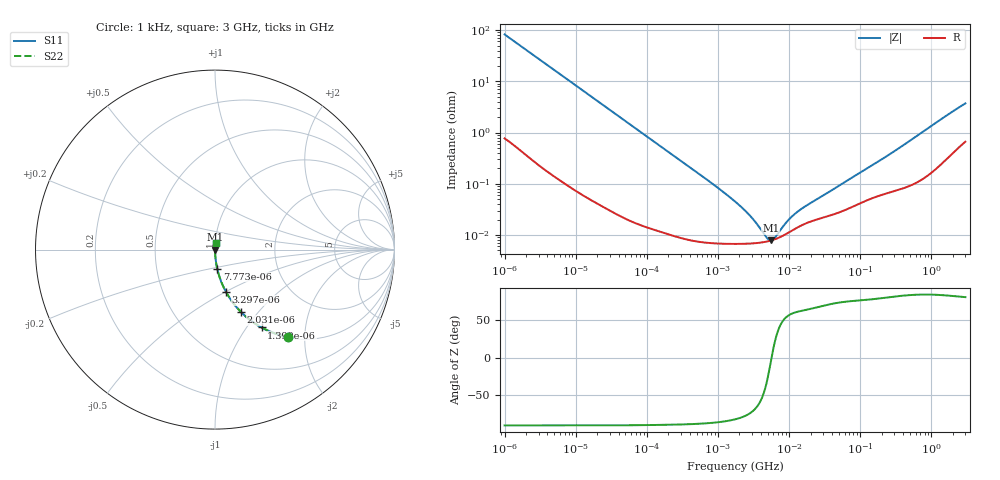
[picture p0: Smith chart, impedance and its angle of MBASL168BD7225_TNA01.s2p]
! MBASL168BD7225_TNA01  S-PARAMETER MODEL  ( Standard Model )
! Model Generated by TAIYO YUDEN Corporation (http://www.ty-top.com)
! Version 1.0
! TAIYO YUDEN Control No. 220601
! Copyright(c) 2015 TAIYO YUDEN CO.,LTD. All Rights Reserved.
! Product Description (link to TY-COMPAS)
! https://ds.yuden.co.jp/TYCOMPAS/or/detail?pn=MBASL168BD7225KTNA01&u=M
! Products Name : Multilayer Ceramic Capacitors
! Characteristics :
!  Capacitance : 2.2 [uF] , Rated Voltage : 10 [V] , TCC : X7T
!  Case Size : 1.6 x 0.8 / 0.063 x 0.031 [mm/inch] , Thickness : 0.8 / 0.031 [mm/inch]
!  (Conditions: Temperature = 25 [degC] , DC Bias Voltage = 0 [V])
! External Node Assignments :
!  1  o---| |---o  2
! GND o---------o GND
! Frequency Range : 1kHz  -  3GHz  [ 401 STEP ]
# MHZ S RI R 50
! Freq[MHz].  S11 Real  S11 Imag  S21 Real  S21 Imag  S12 Real  S12 Imag  S22 Real  S22 Imag
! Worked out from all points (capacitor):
!   401 points, 1 kHz to 3 GHz, reference 50 ohm
!   read as one part in series: C = 1.93 uF near 1.077 kHz
!   lowest |Z| = 7.82 mohm at 5.502 MHz (marker M1)
!   series resonance near 5.662 MHz, so ESL is about 410 pH
!   S11 on the Smith chart (normalised r, x): 1 kHz: 1.02, -1.65; 1.399 kHz: 1.01, -1.18; 2.031 kHz: 1.01, -0.81; 3.297 kHz: 1.00, -0.50; 7.773 kHz: 1.00, -0.21; 3 GHz: 1.01, +0.07
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0.001  0.4044 -0.4861  0.5956 0.4861  0.5956 0.4861  0.4044 -0.4861
0.001399  0.2599 -0.434  0.7401 0.434  0.7401 0.434  0.2599 -0.434
0.002031  0.1443 -0.347  0.8557 0.347  0.8557 0.347  0.1443 -0.347
0.003297  0.0611 -0.2354  0.9389 0.2354  0.9389 0.2354  0.0611 -0.2354
0.007773  0.0122 -0.1056  0.9878 0.1056  0.9878 0.1056  0.0122 -0.1056
0.01216  0.00528 -0.0682  0.9947 0.0682  0.9947 0.0682  0.00528 -0.0682
0.033275  0.000911 -0.0252  0.9991 0.0252  0.9991 0.0252  0.000911 -0.0252
0.147855  0.000151 -0.00571  0.9998 0.00571  0.9998 0.00571  0.000151 -0.00571
0.762639  7.1e-05 -0.0011  0.9999 0.0011  0.9999 0.0011  7.1e-05 -0.0011
1.732051  6.72e-05 -0.000447  0.9999 0.000447  0.9999 0.000447  6.72e-05 -0.000447
2.812335  6.81e-05 -0.000229  0.9999 0.000229  0.9999 0.000229  6.81e-05 -0.000229
4.399271  7.26e-05 -7.68e-05  0.9999 7.68e-05  0.9999 7.68e-05  7.26e-05 -7.68e-05
4.739869  7.4e-05 -5.38e-05  0.9999 5.38e-05  0.9999 5.38e-05  7.4e-05 -5.38e-05
5.502215  7.78e-05 -8.57e-06  0.9999 8.57e-06  0.9999 8.57e-06  7.78e-05 -8.57e-06
6.387174  8.31e-05 3.6e-05  0.9999 -3.6e-05  0.9999 -3.6e-05  8.31e-05 3.6e-05
6.881678  8.66e-05 5.82e-05  0.9999 -5.82e-05  0.9999 -5.82e-05  8.66e-05 5.82e-05
9.273352  0.000107 0.000147  0.9999 -0.000147  0.9999 -0.000147  0.000107 0.000147
11.1738  0.000124 0.000201  0.9999 -0.000201  0.9999 -0.000201  0.000124 0.000201
21.06097  0.000188 0.000398  0.9998 -0.000398  0.9998 -0.000398  0.000188 0.000398
256.0921  0.000686 0.00367  0.9993 -0.00367  0.9993 -0.00367  0.000686 0.00367
1652.1  0.00352 0.0214  0.9965 -0.0214  0.9965 -0.0214  0.00352 0.0214
3000  0.0079 0.036  0.9921 -0.036  0.9921 -0.036  0.0079 0.036
